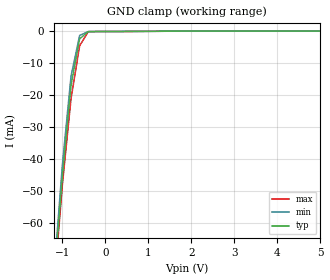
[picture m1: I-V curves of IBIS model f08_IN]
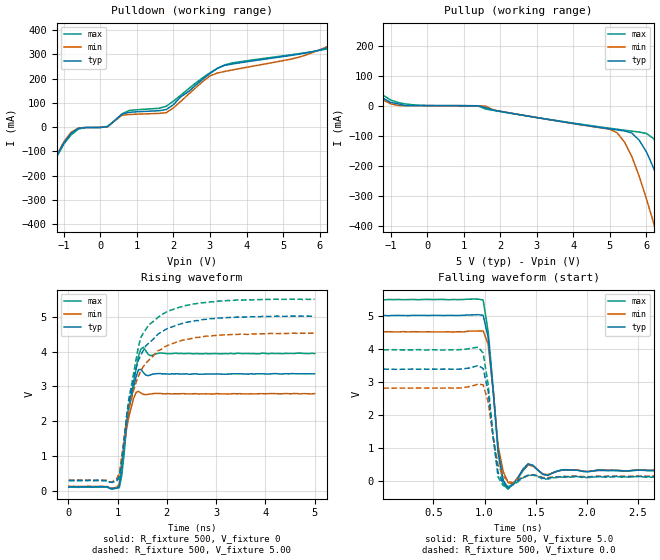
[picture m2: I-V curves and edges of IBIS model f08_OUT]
| TEXAS INSTRUMENTS INCORPORATED
| Standard Linear and Logic Group
| IBIS Model of SN74F08
| QUADRUPLE 2-INPUT POSITIVE-AND GATES
| SOP 14-pin (NS), SSOP 14-pin (DB), SOIC 14-pin (D), PDIP 14-pin (N) packages
[IBIS Ver]   3.2
[Comment Char]  |_char
[File Name]   sn74f08.ibs
[File Rev]   3.1 I_die
[Date]   Nov.01, 2004
[Source]   File originated at Texas Instruments, Inc.
[Notes]   The following is a sample IBIS file for the F08.
   - FILE REV HISTORY
   - 3.1 Re-Release IBIS file on 11/03/04
   - Power clamp data deleted as there is no power-clamp diode.
|   - All test data contained in this file are derived from
|   actual measurements.
|   - File created by Nobuhisa Ohtsubo, SLL Product Engineering.
[Disclaimer] Property of Texas Instruments Incorporated.  Unauthorized
   reproduction and/or distribution is strictly prohibited.
   This product is protected under copyright law.
   Created 2000, (C) Copyright 2000, Texas Instruments Inc.,
   All Rights Reserved.
   UNLESS THERE IS A SIGNED, WRITTEN AGREEMENT TO THE
   CONTRARY, TEXAS INSTRUMENTS () IS PROVIDING THE IBIS
   MODELS  AND WITHOUT ANY WARRANTY, EXPRESSED OR
   IMPLIED.  TI assumes no liability for:
   1) the accuracy of the IBIS models provided to your
   company;
   2) the proper functioning of these IBIS Models in your
   design or for any resulting applications; or
   3) infringement of patents, copyrights or intellectual
   property rights resulting from your use of these IBIS
   models.
   TI provides IBIS Models as a service to our customers.
   You and your company shall not distribute, sell or give
   these models to anyone else without prior written
   permission from TI.
   TI reserves the right to make changes to our products or
   to discontinue any semiconductor product or service
   without notice, and advises our customers to obtain the
   latest version of relevant information to verify, before
   placing orders, that the information being relied on is
   current.
   Please be aware that your receipt and use of the IBIS
   information provided shall serve as acceptance of these
   terms and conditions.  If you do not accept these terms,
   you should return or destroy the IBIS models and any
   other accompanying information immediately.
|   Component f08_NS
[Component]   f08_NS
[Manufacturer]  Texas Instruments, Inc.
[Package]
|   typ   min   max
R_pkg   0.045   0.039   0.054
L_pkg   3.796nH   2.561nH   4.952nH
C_pkg   0.528pF   0.288pF   0.710pF
[Pin]   signal_name   model_name   R_pin   L_pin   C_pin
1   1A   f08_IN   0.047   4.867nH   0.706pF
2   1B   f08_IN   0.051   4.083nH   0.592pF
3   1Y   f08_OUT   0.041   2.915nH   0.376pF
4   2A   f08_IN   0.039   2.561nH   0.288pF
5   2B   f08_IN   0.041   3.101nH   0.430pF
6   2Y   f08_OUT   0.047   4.047nH   0.589pF
7   GND   GND   0.051   4.909nH   0.700pF
8   3Y   f08_OUT   0.045   4.784nH   0.694pF
9   3A   f08_IN   0.054   4.176nH   0.597pF
10   3B   f08_IN   0.039   3.287nH   0.449pF
11   4Y   f08_OUT   0.039   2.586nH   0.294pF
12   4A   f08_IN   0.040   2.802nH   0.371pF
13   4B   f08_IN   0.049   4.080nH   0.593pF
14   VCC   POWER   0.052   4.952nH   0.710pF
|   Component f08_DB
[Component]   f08_DB
[Manufacturer]  Texas Instruments, Inc.
[Package]
|   typ   min   max
R_pkg   0.044   0.041   0.046
L_pkg   3.551nH   3.258nH   3.927nH
C_pkg   0.402pF   0.360pF   0.421pF
[Pin]   signal_name   model_name   R_pin   L_pin   C_pin
1   1A   f08_IN   0.046   3.927nH   0.408pF
2   1B   f08_IN   0.044   3.587nH   0.421pF
3   1Y   f08_OUT   0.041   3.289nH   0.398pF
4   2A   f08_IN   0.042   3.258nH   0.360pF
5   2B   f08_IN   0.041   3.286nH   0.403pF
6   2Y   f08_OUT   0.044   3.586nH   0.421pF
7   GND   GND   0.046   3.927nH   0.408pF
8   3Y   f08_OUT   0.046   3.927nH   0.408pF
9   3A   f08_IN   0.044   3.586nH   0.421pF
10   3B   f08_IN   0.041   3.286nH   0.403pF
11   4Y   f08_OUT   0.043   3.258nH   0.360pF
12   4A   f08_IN   0.041   3.289nH   0.398pF
13   4B   f08_IN   0.044   3.587nH   0.421pF
14   VCC   POWER   0.046   3.927nH   0.408pF
|   Component f08_D
[Component]   f08_D
[Manufacturer]  Texas Instruments, Inc.
[Package]
|   typ   min   max
R_pkg   0.031   0.028   0.034
L_pkg   3.109nH   2.462nH   3.889nH
C_pkg   0.473pF   0.363pF   0.628pF
[Pin]   signal_name   model_name   R_pin   L_pin   C_pin
1   1A   f08_IN   0.033   3.854nH   0.622pF
2   1B   f08_IN   0.032   3.188nH   0.473pF
3   1Y   f08_OUT   0.028   2.462nH   0.377pF
4   2A   f08_IN   0.031   2.596nH   0.363pF
5   2B   f08_IN   0.028   2.521nH   0.372pF
6   2Y   f08_OUT   0.034   3.250nH   0.476pF
7   GND   GND   0.034   3.889nH   0.628pF
8   3Y   f08_OUT   0.034   3.889nH   0.628pF
9   3A   f08_IN   0.034   3.250nH   0.476pF
10   3B   f08_IN   0.028   2.521nH   0.372pF
11   4Y   f08_OUT   0.031   2.596nH   0.364pF
12   4A   f08_IN   0.028   2.462nH   0.377pF
13   4B   f08_IN   0.032   3.188nH   0.473pF
14   VCC   POWER   0.033   3.854nH   0.622pF
|   Component f08_N
[Component]   f08_N
[Manufacturer]   Texas Instruments, Inc.
[Package]
|   typ   min   max
R_pkg   4.500e-02   3.700e-02   6.300e-02
L_pkg   5.407e-09   3.922e-09   6.942e-09
C_pkg   3.890e-13   2.050e-13   6.040e-13
[Pin]   signal_name   model_name   R_pin   L_pin   C_pin
1   1A   f08_IN   6.300e-02   6.942e-09   6.040e-13
2   1B   f08_IN   3.700e-02   6.200e-09   4.060e-13
3   1Y   f08_OUT   4.200e-02   4.389e-09   3.220e-13
4   2A   f08_IN   3.800e-02   3.922e-09   2.050e-13
5   2B   f08_IN   3.900e-02   4.301e-09   2.980e-13
6   2Y   f08_OUT   3.800e-02   5.329e-09   3.560e-13
7   GND   GND   5.300e-02   6.510e-09   5.440e-13
8   3Y   f08_OUT   5.300e-02   6.437e-09   5.390e-13
9   3A   f08_IN   3.900e-02   5.352e-09   3.470e-13
10   3B   f08_IN   4.200e-02   4.473e-09   2.970e-13
11   4Y   f08_OUT   4.400e-02   4.326e-09   2.250e-13
12   4A   f08_IN   4.200e-02   4.295e-09   2.800e-13
13   4B   f08_IN   4.200e-02   6.318e-09   4.180e-13
14   VCC   POWER   6.100e-02   6.900e-09   6.030e-13
| Models and submodels in the file (2): f08_IN (Input), f08_OUT (Output)
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|   Model f08_IN
[Model]   f08_IN
Model_type  Input
Polarity   Non-Inverting
Vinl = 0.8
Vinh = 2.0
| variable   typ   min   max
C_comp   1.33pf   1.00pf   1.66pf
[Temperature Range]   25   0   70
[Voltage Range]   5.0   4.5   5.5
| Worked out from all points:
|   GND clamp passes 1 mA (typ) near -0.47 V on its own axis
[GND Clamp]
|   Voltage   I(typ)   I(min)   I(max)
-5V       -900.4mA   -941.2mA   -843.6mA
-1.2V     -78.63mA   -76.67mA   -81.15mA
-1V       -45.4mA    -41.78mA   -47.94mA
-800mV    -16.94mA   -14.14mA   -21.2mA
-600mV    -2.426mA   -1.372mA   -4.611mA
-400mV    -161.4uA   -149.5uA   -201.7uA
5V        7.996nA    29.34nA    9.3nA
|   Model f08_OUT
[Model]   f08_OUT
Model_type  Output
Polarity   Non-Inverting
Vmeas = 1.5v
Cref = 0pf
| variable   typ   min   max
C_comp   5.8pf   4.35pf   7.25pf
[Temperature Range]   25   0   70
[Voltage Range]   5.0   4.5   5.5
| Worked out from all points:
|   slope of the pulldown table from 0 to 0.75 V, typ, clamps not added: 12.3 ohm
|   slope of the pullup table from 0 to 0.75 V, typ, clamps not added: 16.9 kohm
|   rising waveform, R_fixture 500, V_fixture 0: 20-80 % time 190ps typ, 178ps min, 214ps max; typ from 0.104 V to 3.37 V
|   falling waveform, R_fixture 500, V_fixture 5.0: 20-80 % time 80.1ps typ, 78.9ps min, 84.1ps max; typ from 5.03 V to 0.306 V
|   rising waveform, R_fixture 500, V_fixture 5.00: 20-80 % time 426ps typ, 490ps min, 360ps max; typ from 0.29 V to 5.04 V
|   falling waveform, R_fixture 500, V_fixture 0.0: 20-80 % time 75.1ps typ, 81.3ps min, 81.1ps max; typ from 3.39 V to 0.121 V
[Pulldown]
|   Voltage   I(typ)   I(min)   I(max)
-5V       -1.667A    -1.756A    -1.544A
-2V       -431.5mA   -445.6mA   -411.4mA
-1.2V     -119.6mA   -116.3mA   -123.8mA
-800mV    -25.32mA   -21.21mA   -31.57mA
200mV     2.372mA    1.637mA    3.336mA
800mV     61.22mA    52.08mA    68.96mA
1.8V      72.21mA    59.41mA    85.9mA
3V        220.9mA    210.5mA    223.7mA
3.4V      254.1mA    229.1mA    256.1mA
5.6V      304.5mA    295.3mA    306mA
7.4V      405.7mA    420.7mA    388.6mA
10V       586mA      628.4mA    553.4mA
[Pullup]
|   Voltage   II(typ)   I(min)   I(max)
-5V       260.7mA    231.8mA    259.3mA
-1V       10.68mA    6.098mA    18.58mA
1.6V      -7.358mA   -1.67mA    -11.18mA
5V        -77.58mA   -78.79mA   -75.47mA
5.4V      -84.39mA   -121.6mA   -81.92mA
5.8V      -114.8mA   -234.9mA   -88.01mA
6.2V      -209.3mA   -392.7mA   -110.4mA
6.4V      -277.3mA   -477.3mA   -144.3mA
6.8V      -429.9mA   -622.2mA   -246.9mA
7.2V      -578.7mA   -774.9mA   -382.9mA
7.4V      -653.8mA   -851.3mA   -454.8mA
10V       -1.63A     -1.844A    -1.364A
[Ramp]
| variable   typ   min   max
dV/dt_r   1.910E+00/1.880E-09  1.560E+00/1.820E-09  2.270E+00/2.140E-09
dV/dt_f   2.850E+00/7.800E-10  2.540E+00/7.600E-10  3.140E+00/8.200E-10
R_load = 500
[Rising Waveform]
R_fixture = 500
V_fixture = 0
|   Time   V(typ)   V(min)   V(max)
9.766ps   104.3mV    126.5mV    101.1mV
1.035ns   136.4mV    193.7mV    85.44mV
1.084ns   607.8mV    766.1mV    426.9mV
1.182ns   1.912V     1.775V     1.872V
1.23ns    2.375V     2.134V     2.434V
1.328ns   2.993V     2.665V     3.14V
1.426ns   3.485V     2.858V     3.885V
1.523ns   3.403V     2.772V     4.128V
1.67ns    3.332V     2.782V     3.888V
5ns       3.365V     2.793V     3.947V
[Falling Waveform]
R_fixture = 500
V_fixture = 5.0
V_fixture_min = 4.5
V_fixture_max = 5.5
C_fixture = 0pf
L_fixture = 0nH
|   Time   V(typ)   V(min)   V(max)
9.766ps   5.025V     4.525V     5.494V
986.3ps   5.026V     4.552V     5.491V
1.035ns   4.361V     4.152V     4.537V
1.133ns   895mV      1.052V     862.6mV
1.182ns   20.13mV    287.5mV    -115.7mV
1.23ns    -222.7mV   -55.66mV   -255.8mV
1.279ns   -118.8mV   -102.2mV   -88.31mV
1.426ns   516.4mV    488.6mV    479.8mV
1.621ns   161.2mV    187.6mV    173.1mV
5ns       305.6mV    302mV      278.1mV
[Rising Waveform]
R_fixture = 500
V_fixture = 5.00
V_fixture_min = 4.50
V_fixture_max = 5.50
C_fixture = 0pf
L_fixture = 0nH
|   Time
9.766ps   290mV      302mV      287.2mV
888.7ps   235.6mV    255.4mV    240.3mV
1.035ns   412.9mV    501.4mV    358.1mV
1.084ns   841.4mV    986.4mV    679.8mV
1.23ns    2.589V     2.351V     2.661V
1.426ns   3.769V     3.303V     4.163V
1.621ns   4.23V      3.74V      4.746V
1.865ns   4.546V     4.052V     5.037V
2.793ns   4.933V     4.446V     5.417V
5ns       5.037V     4.534V     5.506V
[Falling Waveform]
R_fixture = 500
V_fixture = 0.0
|   Time
9.766ps   3.391V     2.812V     3.976V
937.5ps   3.501V     2.936V     4.059V
986.3ps   3.408V     2.913V     3.879V
1.035ns   2.718V     2.397V     2.926V
1.084ns   1.323V     1.329V     1.332V
1.133ns   237.2mV    467.5mV    102.3mV
1.182ns   -79.56mV   147mV      -149.4mV
1.279ns   -110.3mV   -63mV      -125mV
1.475ns   180.3mV    186.8mV    170.9mV
5ns       121.1mV    124.2mV    104.8mV
